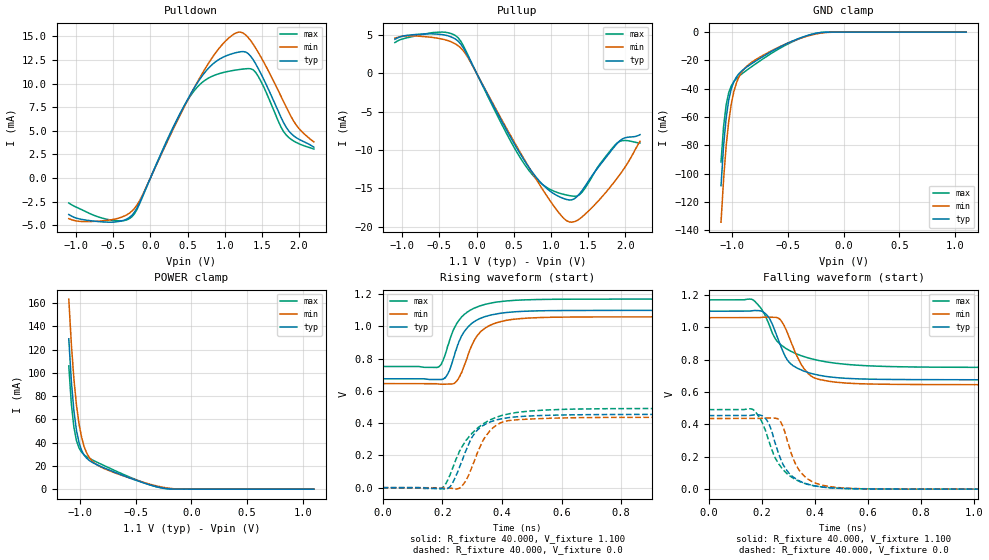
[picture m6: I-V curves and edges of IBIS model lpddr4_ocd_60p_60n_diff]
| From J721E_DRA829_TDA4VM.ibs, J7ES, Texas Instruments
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|   Model lpddr4_ocd_60p_60n_diff
[Model] lpddr4_ocd_60p_60n_diff
Model_type I/O
Polarity   Non-Inverting
Enable   Active-High
Vinl =  0.113V
Vinh =  0.253V
Vmeas =  0.183V
C_comp   1.892pF   1.705pF   2.160pF
[Model Spec]
Vinh   0.253V   0.247V   0.265V
Vinl   0.113V   0.107V   0.125V
Vmeas   0.183V   0.176V   0.195V
[Temperature Range]   25.000   0.125k   -40.000
[Voltage Range]   1.100V   1.060V   1.170V
[Pullup Reference]   1.100V   1.060V   1.170V
[Pulldown Reference]   0.0V   0.0V   0.0V
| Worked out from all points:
|   slope of the pulldown table from 0 to 0.165 V, typ, clamps not added: 56.5 ohm
|   slope of the pullup table from 0 to 0.165 V, typ, clamps not added: 53.4 ohm
|   GND clamp passes 1 mA (typ) near -0.25 V on its own axis
|   POWER clamp passes 1 mA (typ) near -0.26 V on its own axis
|   rising waveform, R_fixture 40.000, V_fixture 1.100: 20-80 % time 65.6ps typ, 66.3ps min, 70.4ps max; typ from 0.676 V to 1.1 V
|   rising waveform, R_fixture 40.000, V_fixture 0.0: 20-80 % time 71.5ps typ, 67.3ps min, 105ps max; typ from 0 V to 0.455 V
|   falling waveform, R_fixture 40.000, V_fixture 1.100: 20-80 % time 79.9ps typ, 73.8ps min, 123ps max; typ from 1.1 V to 0.676 V
|   falling waveform, R_fixture 40.000, V_fixture 0.0: 20-80 % time 70.8ps typ, 68.6ps min, 86.9ps max; typ from 0.455 V to 0 V
[Pulldown]
|Voltage   I(typ)   I(min)   I(max)
-1.1V     -3.87mA    -4.304mA   -2.646mA
-590mV    -4.675mA   -4.496mA   -4.367mA
-249mV    -3.947mA   -3.505mA   -4.103mA
-113mV    -2.039mA   -1.898mA   -2.107mA
329mV     5.685mA    5.544mA    5.764mA
567mV     9.253mA    9.238mA    9.025mA
839mV     12.07mA    12.84mA    10.81mA
1.179V    13.33mA    15.45mA    11.47mA
1.384V    12.52mA    14.17mA    11.46mA
1.826V    5.392mA    7.543mA    4.569mA
1.996V    4.117mA    5.272mA    3.639mA
2.2V      3.262mA    3.828mA    3.066mA
[Pullup]
|Voltage   I(typ)   I(min)   I(max)
-1.1V     4.426mA    4.571mA    4.004mA
-590mV    5.136mA    4.667mA    5.303mA
-249mV    4.188mA    3.596mA    4.628mA
-113mV    2.15mA     1.986mA    2.301mA
397mV     -7.294mA   -7.066mA   -7.74mA
669mV     -11.76mA   -11.68mA   -12.2mA
941mV     -14.99mA   -15.92mA   -14.87mA
1.247V    -16.52mA   -19.38mA   -15.95mA
1.418V    -15.32mA   -18.75mA   -15.53mA
1.656V    -12.04mA   -16.46mA   -11.89mA
1.894V    -9.129mA   -13.66mA   -9.086mA
2.2V      -8.007mA   -8.873mA   -9.081mA
[GND_clamp]
|Voltage   I(typ)   I(min)   I(max)
-1.1V     -108.4mA   -134.2mA   -91.64mA
-1.077V   -80.17mA   -103.9mA   -66.63mA
-1.054V   -60.68mA   -80.47mA   -51.43mA
-1.031V   -48.01mA   -63.16mA   -42.83mA
-1.008V   -40.05mA   -50.75mA   -37.96mA
-985mV    -35.04mA   -42.04mA   -34.98mA
-940mV    -29.42mA   -31.64mA   -31.22mA
-894mV    -26.11mA   -26.16mA   -28.35mA
-848mV    -23.5mA    -22.73mA   -25.7mA
-527mV    -8.739mA   -8.686mA   -9.514mA
-229mV    -630.6uA   -1.042mA   -565.5uA
1.1V      0A         0A         0A
[POWER_clamp]
|Voltage   I(typ)   I(min)   I(max)
-1.1V     129.2mA    163.4mA    105.9mA
-1.077V   92.86mA    124.8mA    73.4mA
-1.054V   67.3mA     94.73mA    53.17mA
-1.031V   50.48mA    72.25mA    41.67mA
-1.008V   39.92mA    56.03mA    35.37mA
-985mV    33.38mA    44.6mA     31.76mA
-963mV    29.31mA    36.69mA    29.53mA
-917mV    24.75mA    27.38mA    26.61mA
-871mV    22.09mA    22.57mA    24.31mA
-619mV    11.98mA    11.76mA    13.12mA
-229mV    602.6uA    1.183mA    400.7uA
1.1V      0A         0A         0A
[Ramp]
| variable   typ   min   max
dV/dt_r   0.273/71.076p   0.262/67.341p   0.295/0.106n
dV/dt_f   0.255/79.379p   0.249/72.948p   0.251/0.122n
R_load = 40.000
[Rising Waveform]
R_fixture= 40.000
V_fixture= 1.100
V_fixture_min= 1.060
V_fixture_max= 1.170
|time   V(typ)   V(min)   V(max)
0s        675.6mV    645.6mV    752mV
186ps     671.4mV    643.3mV    747.5mV
197ps     671mV      641.7mV    767.1mV
215ps     694.1mV    642.4mV    855.4mV
239ps     810.2mV    646.2mV    986mV
272ps     964.7mV    750.1mV    1.073V
306ps     1.028V     910.8mV    1.113V
328ps     1.051V     966.9mV    1.129V
441ps     1.091V     1.045V     1.162V
3ns       1.1V       1.06V      1.17V
[Rising Waveform]
R_fixture= 40.000
V_fixture= 0.0
V_fixture_min= 0.0
V_fixture_max= 0.0
|time   V(typ)   V(min)   V(max)
0s        295.9uV    499uV      527.8uV
196ps     -4.908mV   -3.183mV   -5.786mV
226ps     5.271mV    -2.568mV   79.18mV
254ps     111.3mV    -6.337mV   208.7mV
283ps     246.5mV    56.86mV    300.9mV
309ps     340.7mV    173.6mV    355.5mV
340ps     389mV      304.3mV    399.9mV
368ps     412.7mV    368.5mV    426.9mV
495ps     445.2mV    426.1mV    475.6mV
3ns       455mV      437mV      491.8mV
[Falling Waveform]
R_fixture= 40.000
V_fixture= 1.100
V_fixture_min= 1.060
V_fixture_max= 1.170
|time   V(typ)   V(min)   V(max)
0s        1.1V       1.06V      1.17V
167ps     1.104V     1.06V      1.171V
217ps     1.081V     1.063V     1.057V
261ps     931.2mV    1.059V     909.4mV
302ps     786.5mV    945.2mV    859.3mV
332ps     749.8mV    824.4mV    835.8mV
374ps     721.6mV    715.7mV    812mV
488ps     688.7mV    660mV      776.7mV
855ps     676.7mV    646.4mV    754mV
3ns       675.6mV    645.6mV    752mV
[Falling Waveform]
R_fixture= 40.000
V_fixture= 0.0
V_fixture_min= 0.0
V_fixture_max= 0.0
|time   V(typ)   V(min)   V(max)
0s        455mV      437mV      491.8mV
167ps     458.7mV    437mV      493.1mV
194ps     458mV      437.8mV    437.1mV
219ps     427.2mV    440.5mV    339.3mV
262ps     228mV      434.2mV    162.9mV
294ps     116.6mV    314.5mV    98.15mV
339ps     54.06mV    123.2mV    50.18mV
375ps     30.28mV    61.37mV    29.24mV
435ps     12.09mV    22.74mV    12.46mV
3ns       295.8uV    498.7uV    527.8uV
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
